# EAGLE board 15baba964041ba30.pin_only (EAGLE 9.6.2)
REV: A

Size 104.01 x 69.85 mm. Coordinates in mm from the lower left corner, seen from the top.
Outline: 0,69.85 0,0 104.01,0 104.01,69.85 0,69.85
Copper layers (1*16): Top 0.035mm / dielectric 1.5mm / Bottom 0.035mm
Design rules "adafruit 8-8": minimum track width 6mil, minimum drill 15.5mil, track to track 8mil, track to pad 8mil, pad to pad 8mil, via to via 8mil, smd to smd 8mil, copper to edge 10mil, drill to drill 8mil, minimum pad ring 10mil, minimum via ring 8mil, stop-mask expansion 2mil, vias tented up to drill 20mil, thermal gap 10mil
Net classes: 1 power: width 0.254 mm

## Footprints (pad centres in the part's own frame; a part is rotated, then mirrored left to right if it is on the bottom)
0805-NO = smd 1.24 x 1.5: 1 -0.95,0; 2 0.95,0
PICOWBELL_DUALSMT = smd 1.524 x 2.032: S1 -24.13,-12.889; S2 -24.13,-7.555; S3 -21.59,-12.889; S4 -21.59,-7.555; S37 21.59,-12.889; S38 21.59,-7.555; S39 24.13,-12.889; S40 24.13,-7.555; S41 24.13,12.889; S42 24.13,7.555; S43 21.59,12.889; S44 21.59,7.555; S77 -21.59,7.555; S78 -21.59,12.889; S79 -24.13,7.555; S80 -24.13,12.889 | smd 1.524 x 3.048: S5 -19.05,-12.381; S6 -19.05,-8.063; S7 -16.51,-12.381; S8 -16.51,-8.063; S9 -13.97,-12.381; S10 -13.97,-8.063; S11 -11.43,-12.381; S12 -11.43,-8.063; S13 -8.89,-12.381; S14 -8.89,-8.063; S15 -6.35,-12.381; S16 -6.35,-8.063; S17 -3.81,-12.381; S18 -3.81,-8.063; S19 -1.27,-12.381; S20 -1.27,-8.063; S21 1.27,-12.381; S22 1.27,-8.063; S23 3.81,-12.381; S24 3.81,-8.063; S25 6.35,-12.381; S26 6.35,-8.063; S27 8.89,-12.381; S28 8.89,-8.063; S29 11.43,-12.381; S30 11.43,-8.063; S31 13.97,-12.381; S32 13.97,-8.063; S33 16.51,-12.381; S34 16.51,-8.063; S35 19.05,-12.381; S36 19.05,-8.063; S45 19.05,8.063; S46 19.05,12.381; S47 16.51,8.063; S48 16.51,12.381; S49 13.97,8.063; S50 13.97,12.381; S51 11.43,8.063; S52 11.43,12.381; S53 8.89,8.063; S54 8.89,12.381; S55 6.35,8.063; S56 6.35,12.381; S57 3.81,8.063; S58 3.81,12.381; S59 1.27,8.063; S60 1.27,12.381; S61 -1.27,8.063; S62 -1.27,12.381; S63 -3.81,8.063; S64 -3.81,12.381; S65 -6.35,8.063; S66 -6.35,12.381; S67 -8.89,8.063; S68 -8.89,12.381; S69 -11.43,8.063; S70 -11.43,12.381; S71 -13.97,8.063; S72 -13.97,12.381; S73 -16.51,8.063; S74 -16.51,12.381; S75 -19.05,8.063; S76 -19.05,12.381 | hole 2: -22.86,10.222; 22.86,10.222; 22.86,-10.098; -22.86,-10.098
JST_SH4 = smd 0.6 x 1.55: 1 -1.5,2.006; 2 -0.5,2.006; 3 0.5,2.006; 4 1.5,2.006 | smd 1.2 x 1.8: MT1 -2.8,-1.894; MT2 2.8,-1.894
FIDUCIAL_1MM = smd 1 x 1: 1 0,0
SO08-SKINNYPADS = smd 0.66 x 1.524: 1 -1.905,-2.973; 2 -0.635,-2.973; 3 0.635,-2.973; 4 1.905,-2.973; 5 1.905,2.973; 6 0.635,2.973; 7 -0.635,2.973; 8 -1.905,2.973
2X20_SMT_MALE = smd 1.524 x 2.032: 1 -24.13,-2.667; 2 -24.13,2.667; 3 -21.59,-2.667; 4 -21.59,2.667; 37 21.59,-2.667; 38 21.59,2.667; 39 24.13,-2.667; 40 24.13,2.667 | smd 1.524 x 3.048: 5 -19.05,-2.159; 6 -19.05,2.159; 7 -16.51,-2.159; 8 -16.51,2.159; 9 -13.97,-2.159; 10 -13.97,2.159; 11 -11.43,-2.159; 12 -11.43,2.159; 13 -8.89,-2.159; 14 -8.89,2.159; 15 -6.35,-2.159; 16 -6.35,2.159; 17 -3.81,-2.159; 18 -3.81,2.159; 19 -1.27,-2.159; 20 -1.27,2.159; 21 1.27,-2.159; 22 1.27,2.159; 23 3.81,-2.159; 24 3.81,2.159; 25 6.35,-2.159; 26 6.35,2.159; 27 8.89,-2.159; 28 8.89,2.159; 29 11.43,-2.159; 30 11.43,2.159; 31 13.97,-2.159; 32 13.97,2.159; 33 16.51,-2.159; 34 16.51,2.159; 35 19.05,-2.159; 36 19.05,2.159 | hole 2: -22.86,0; 22.86,0
1X12_OVAL = drill 1 pad 1.676 long: 1 -13.97,0; 2 -11.43,0; 3 -8.89,0; 4 -6.35,0; 5 -3.81,0; 6 -1.27,0; 7 1.27,0; 8 3.81,0; 9 6.35,0; 10 8.89,0; 11 11.43,0; 12 13.97,0
SOT23-WIDE = smd 1 x 1.2: 1 -0.95,-1; 2 0.95,-1; 3 0,1
0603-NO = smd 1.075 x 1: 1 -0.85,0; 2 0.85,0
PS12 = drill 1 pad 2.54: P$1 -2.5,0; P$2 2.5,0
B3F-40XX-SMT = smd 2 x 2: P$1 -7,2.5; P$2 7,2.5; P$3 -7,-2.5; P$4 7,-2.5 | hole 1.803: 0,-4.496; 0,4.496
EG1390 = smd 1 x 1.5: O1 -2.5,2.8; O2 -2.5,-2.8; P1 0,2.8; P2 0,-2.8; S1 2.5,2.8; S2 2.5,-2.8 | hole 1: 1.5,0; -1.5,0
TFT_1.9IN_170X320_30P_SS = smd 0.28 x 1.25: 1 -7.25,1.236; 2 -6.75,1.236; 3 -6.25,1.236; 4 -5.75,1.236; 5 -5.25,1.236; 6 -4.75,1.236; 7 -4.25,1.236; 8 -3.75,1.236; 9 -3.25,1.236; 10 -2.75,1.236; 11 -2.25,1.236; 12 -1.75,1.236; 13 -1.25,1.236; 14 -0.75,1.236; 15 -0.25,1.236; 16 0.25,1.236; 17 0.75,1.236; 18 1.25,1.236; 19 1.75,1.236; 20 2.25,1.236; 21 2.75,1.236; 22 3.25,1.236; 23 3.75,1.236; 24 4.25,1.236; 25 4.75,1.236; 26 5.25,1.236; 27 5.75,1.236; 28 6.25,1.236; 29 6.75,1.236; 30 7.25,1.236 | smd 2.3 x 4: MNT1 -8.92,-1.02; MNT2 9.42,-1.02
SMT_NUT_3MM = drill 4.25 pad 4.572: P$1 0,0
MOUNTINGHOLE_3.0_PLATEDTHIN = drill 3 pad 3.6: P$1 0,0
TRIMPOT_BOURNS_TC33X-2 = smd 1.2 x 1.2: 1 -1,-1.8; 3 1,-1.8 | smd 1.6 x 1.5: 2 0,1.45
USB_HOST-SMT = smd 1 x 3: D+ 1,0.495; D- -1,0.495; GND 3.5,0.495; VBUS -3.5,0.495 | smd 2.2 x 6: MT1 -7.1,-2.413; MT2 7.1,-2.413 | hole 1.5: -2.5,-3.863; 2.5,-3.863
MICROSD = smd 0.7 x 1.5: 1 1.761,-3.147; 2 0.661,-2.747; 3 -0.439,-3.147; 4 -1.539,-3.547; 5 -2.639,-3.147; 6 -3.739,-3.547; 7 -4.839,-3.147; 8 -5.939,-3.147 | smd 1.8 x 1.4: CD1 -5.239,7.053; CD2 0.38,7.053 | smd 1.4 x 1.9: MT1 -6.839,-6.047; MT2 6.361,-6.947
FPC_0.5MM_18PIN = smd 0.25 x 1.4: 1 4.25,1.154; 2 3.75,1.154; 3 3.25,1.154; 4 2.75,1.154; 5 2.25,1.154; 6 1.75,1.154; 7 1.25,1.154; 8 0.75,1.154; 9 0.25,1.154; 10 -0.25,1.154; 11 -0.75,1.154; 12 -1.25,1.154; 13 -1.75,1.154; 14 -2.25,1.154; 15 -2.75,1.154; 16 -3.25,1.154; 17 -3.75,1.154; 18 -4.25,1.154 | smd 1.8 x 3.5: SUPPORT1 -5.8,-1.152; SUPPORT2 5.8,-1.152

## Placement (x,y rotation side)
C1  10uF  [0805-NO]  87.63,43.69 270 top
C2  10uF  [0805-NO]  66.17,33.27 270 top
C3  10uF  [0805-NO]  91.95,34.29 180 top
C4  10uF  [0805-NO]  87.5,52.07 270 top
C5  10uF  [0805-NO]  16.76,57.91 180 top
C6  10uF  [0805-NO]  52.58,57.15 180 top
C7  10uF  [0805-NO]  24.64,9.4 180 top
C8  10uF  [0805-NO]  90.17,41.15 90 top
C9  10uF  [0805-NO]  11.68,29.46 90 top
CB1  PICOWBELL_DUALSMT  [PICOWBELL_DUALSMT]  31.75,53.34 0 top
CONN1  STEMMA_I2C_QT  [JST_SH4]  94.74,66.67 180 top
FID1  FIDUCIAL_1MM  [FIDUCIAL_1MM]  3.43,7.62 0 top
FID2  FIDUCIAL_1MM  [FIDUCIAL_1MM]  2.92,61.09 0 top
FID3  FIDUCIAL_1MM  [FIDUCIAL_1MM]  101.73,7.49 0 top
IC1  WS2811-SOP8  [SO08-SKINNYPADS]  70.1,32.51 0 top
JP1  16x2 LCD  [2X20_SMT_MALE]  38.73,34.04 0 top
JP8  [1X12_OVAL]  98.55,48.26 270 top
Q1  DMG34x5  [SOT23-WIDE]  84.58,51.82 0 top
Q2  DMG34x5  [SOT23-WIDE]  84.84,44.2 0 top
Q3  BSS138  [SOT23-WIDE]  80.77,51.56 0 top
Q4  BSS138  [SOT23-WIDE]  81.03,43.43 0 top
Q5  BSS138  [SOT23-WIDE]  24.64,14.86 0 top
R1  10K  [0603-NO]  90.81,52.7 0 top
R2  10K  [0603-NO]  90.81,51.18 180 top
R3  10K  [0603-NO]  84.58,49.28 0 top
R4  10K  [0603-NO]  84.58,41.66 0 top
R5  10K  [0603-NO]  57.15,57.66 90 top
R6  27  [0603-NO]  25.4,17.65 0 top
R7  27  [0603-NO]  25.4,19.18 0 top
R8  27  [0603-NO]  25.4,20.7 0 top
R9  27  [0603-NO]  25.4,22.23 0 top
SP1  SPEAKER/PS12  [PS12]  64.39,44.45 270 top
SW1  12mm SMT  [B3F-40XX-SMT]  93.47,11.05 90 top
SW2  DPDT SLIDE  [EG1390]  74.42,42.29 180 top
TFT1  DISP_LCD_ST7789_1.9IN_SS  [TFT_1.9IN_170X320_30P_SS]  30.61,16.13 90 top
TP1  SEWTAP_SMTNUTM3  [SMT_NUT_3MM]  9.14,4.19 0 top
TP2  SEWTAP_SMTNUTM3  [SMT_NUT_3MM]  9.14,35.31 0 top
TP3  SEWTAP_SMTNUTM3  [SMT_NUT_3MM]  84.07,35.31 0 top
TP4  SEWTAP_SMTNUTM3  [SMT_NUT_3MM]  84.07,4.32 0 top
U$7  MOUNTINGHOLE3.0THIN  [MOUNTINGHOLE_3.0_PLATEDTHIN]  100.84,66.55 0 top
U$8  MOUNTINGHOLE3.0THIN  [MOUNTINGHOLE_3.0_PLATEDTHIN]  3.17,66.67 0 top
U$9  MOUNTINGHOLE3.0THIN  [MOUNTINGHOLE_3.0_PLATEDTHIN]  3.17,3.17 0 top
U$10  MOUNTINGHOLE3.0THIN  [MOUNTINGHOLE_3.0_PLATEDTHIN]  100.84,3.05 0 top
U$13  [PCBFEAT-REV-040]  2.16,49.4 90 top
VR1  10K Trimmer  [TRIMPOT_BOURNS_TC33X-2]  3.3,12.06 0 top
X1  USB A  [USB_HOST-SMT]  82.8,56.52 180 top
X2  MicroSD  [MICROSD]  65.79,60.96 180 top
X3  TESTER_PROGCABLE_FLIP  [FPC_0.5MM_18PIN]  100.2,25.15 90 top

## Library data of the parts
C1 C2 C4 = microbuilder; LCSC: C15850
C3 C5-C9 JP8 R1-R5 SP1 = microbuilder
CB1 = adafruit_micro
CONN1 = adafruit_electromech; LCSC: C2845363
FID1-FID3 = microbuilder; BOM: EXCLUDE
IC1 = adafruit; LCSC: C114581
JP1 = adafruit_electromech; LCSC: C2685112
Q1 Q2 = microbuilder; LCSC: C133233; ROT: 270
Q3-Q5 = microbuilder; LCSC: C435876; ROT: 270
R6-R9 = microbuilder; LCSC: C25190
SW1 = adafruit_electromech; LCSC: C455220
SW2 = adafruit_electromech; LCSC: C318999
TFT1 = adafruit_display; LCSC: C262671
TP1-TP4 = adafruit_electromech; FORCETHM: 1; LCSC: C2916369
U$7-U$10 = adafruit_electromech; BOM: EXCLUDE
U$13 = microbuilder; REV: A
VR1 = microbuilder; LCSC: C719176; ROT: 270
X1 = adafruit_electromech; LCSC: C283549
X2 = adafruit_electromech; JLC_ROTATION: 90; LCSC: C125617
X3 = adafruit_electromech; LCSC: C2856802

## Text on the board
tPlace: SDA | SCL | RP2040 Pico | Vbat | Vmeas | USB / Host | MicroSD | GND | Reset | RX/TX | SWDIO | SWCLK | #28 | RXD | TXD | 3V | RP2040 Tester Brains | 18pin Prog / FPC Cable | 16x2 RGB | 10K | LCD / Contrast | Reset

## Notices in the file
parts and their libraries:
microbuilder: This work is placed in the public domain, and may be freely used for commercial and non-commercial work with the following conditions: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
